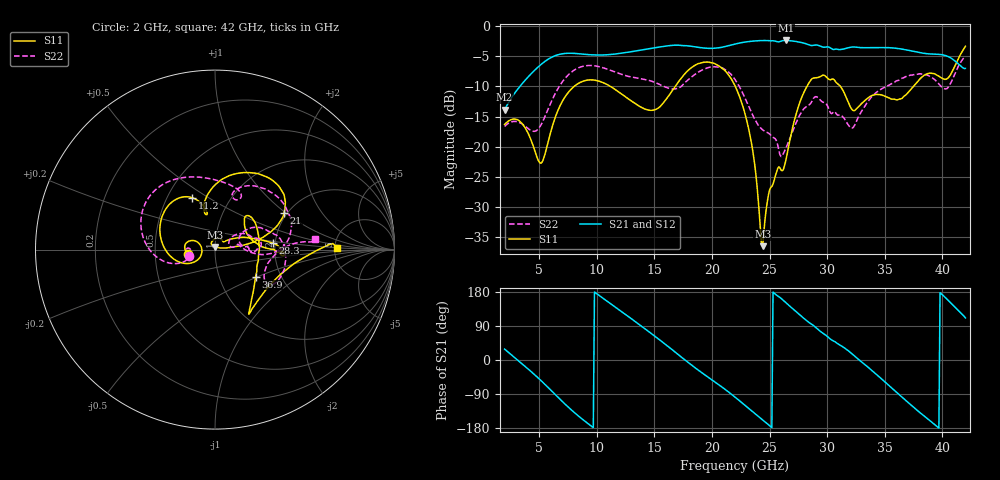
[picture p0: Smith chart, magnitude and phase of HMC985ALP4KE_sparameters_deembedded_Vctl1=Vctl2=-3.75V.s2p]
!s2p File: Measurements: S11, S21, S12, S22
# GHz S dB R 50.0
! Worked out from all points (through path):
!   401 points, 2 GHz to 42 GHz, reference 50 ohm
!   highest |S21| = -2.40 dB at 26.4 GHz (marker M1); lowest = -13.9 dB at 2 GHz (marker M2)
!   lowest |S11| = -36.5 dB at 24.4 GHz (marker M3), VSWR 1.03, Z = 50.1 + j1.5 ohm
!   |S11| at or under -10 dB: start of sweep to 8.041 GHz; 22.02 GHz to 28.25 GHz (6.223 GHz wide, 24.8 % of centre); 31.14 GHz to 37.48 GHz (6.337 GHz wide, 18.5 % of centre)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
!   |S22| runs from -21.6 to -5.0 dB; largest |S21 - S12| = 0.00069
!   S11 on the Smith chart (normalised r, x): 2 GHz: 0.74, -0.04; 11.2 GHz: 0.67, +0.43; 21 GHz: 1.93, +0.98; 28.3 GHz: 1.94, +0.16; 36.9 GHz: 1.49, -0.49; 42 GHz: 5.21, +0.22
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2  -16.31 -170.6  -13.87 28.8  -13.87 28.8  -16.65 -165.5
3.4  -15.93 164.8  -9.84 -7.2  -9.84 -7.2  -16.10 177.7
5.2  -22.68 -172.4  -6.32 -55.5  -6.32 -55.5  -16.24 -162.5
6.8  -13.26 -162.3  -4.69 -103.3  -4.69 -103.3  -9.85 -171.8
8.7  -9.23 149.5  -4.65 -155.0  -4.65 -155.0  -6.74 150.4
11.2  -10.03 113.6  -4.73 148.5  -4.73 148.5  -7.35 109.4
13.5  -13.05 102.5  -4.11 97.8  -4.11 97.8  -8.63 77.2
15.4  -13.51 105.7  -3.51 54.4  -3.51 54.4  -9.63 63.7
17.9  -7.41 77.6  -3.29 -5.6  -3.29 -5.6  -8.97 70.5
21  -7.18 28.1  -3.47 -74.3  -3.47 -74.3  -7.04 16.7
22  -9.90 17.3  -3.00 -97.9  -3.00 -97.9  -8.86 0.2
23.4  -19.11 8.1  -2.54 -132.8  -2.54 -132.8  -14.20 -3.9
24.4  -36.46 86.7  -2.42 -158.0  -2.42 -158.0  -17.22 9.6
25  -27.18 118.3  -2.45 -173.4  -2.45 -173.4  -17.88 12.6
26.4  -22.36 39.1  -2.40 151.7  -2.40 151.7  -20.28 33.1
28.3  -9.82 6.5  -3.04 101.9  -3.04 101.9  -13.20 18.1
28.7  -8.71 0.5  -3.24 93.4  -3.24 93.4  -12.36 15.3
32.4  -13.99 30.7  -3.49 9.8  -3.49 9.8  -16.38 26.7
35.4  -11.93 15.3  -3.60 -68.2  -3.60 -68.2  -9.78 17.3
36.9  -11.31 -33.7  -3.98 -108.7  -3.97 -108.8  -8.33 4.3
39.7  -8.32 -55.8  -4.71 -179.7  -4.71 -179.7  -9.62 -32.6
42  -3.37 1.0  -7.03 111.0  -7.04 111.0  -5.04 6.2
